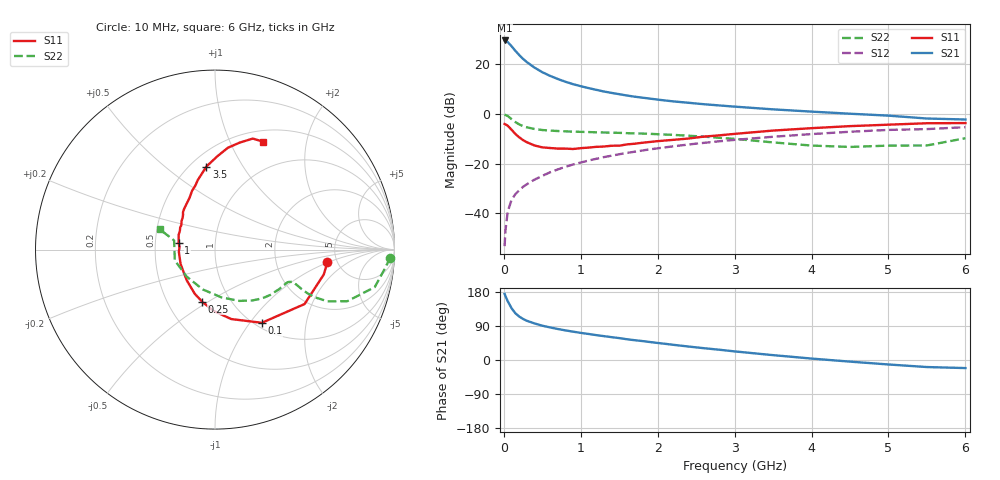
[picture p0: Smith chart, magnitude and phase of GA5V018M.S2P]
! Infineon Technologies  Discrete & RF Semiconductors
! BF775
! Si NPN RF Bipolar Junction Transistor in SOT23
! VCE = 5 V  IC = 18 mA
! Common Emitter S-Parameters:  May  1996
# GHz  S  MA  R  50
!  f  S11  S21  S12  S22
! GHz  MAG  ANG  MAG  ANG  MAG  ANG  MAG  ANG
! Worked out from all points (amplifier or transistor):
!   36 points, 10 MHz to 6 GHz, reference 50 ohm
!   highest |S21| = 29.6 dB at 10 MHz (marker M1)
!   |S21| within 3 dB of that: start of sweep to 118.7 MHz
!   unconditionally stable (mu >= 1): 437.1 MHz to 2.916 GHz
!   at 250 MHz: K = 0.82, MSG = 25.7 dB, |S12| = -29.3 dB
!   at 1.4 GHz: K = 1.10, MAG = 10.7 dB, |S12| = -16.8 dB
!   at 6 GHz: K = 0.93, MSG = 1.5 dB, |S12| = -5.3 dB
!   S11 on the Smith chart (normalised r, x): 10 MHz: 4.16, -0.99; 100 MHz: 1.07, -1.14; 250 MHz: 0.74, -0.47; 1 GHz: 0.66, +0.05; 3.5 GHz: 0.60, +0.71; 6 GHz: 0.63, +1.34
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0.01  0.6304 -6.5  30.22 174.5  0.0022 85.6  0.9769 -2.6
0.02  0.6217 -12.9  29.92 169.3  0.0044 83.9  0.9576 -5.6
0.05  0.5839 -31.3  28.12 155.3  0.0108 77.2  0.9143 -13.2
0.1  0.4841 -57.4  23.17 136.8  0.0188 70.0  0.7915 -21.3
0.15  0.3972 -76.9  18.72 123.3  0.0245 65.6  0.6903 -24.7
0.2  0.3408 -91.6  15.39 114.7  0.0293 65.2  0.6193 -25.5
0.25  0.2986 -103.9  12.88 108.3  0.0344 66.0  0.5713 -25.3
0.3  0.2708 -114.6  11.06 103.4  0.0388 67.2  0.5401 -24.8
0.4  0.2328 -132.4  8.572 96.4  0.0481 68.3  0.5003 -23.5
0.5  0.2138 -146.1  6.946 90.5  0.0571 69.4  0.477 -22.8
0.6  0.2075 -157.5  5.872 86.0  0.0672 69.5  0.4648 -22.8
0.7  0.2019 -167.4  5.082 81.9  0.0768 69.9  0.4558 -23.2
0.8  0.2018 -176.8  4.468 78.2  0.0867 69.4  0.4485 -23.7
1  0.2061 169.5  3.631 71.6  0.106 68.6  0.4385 -25.3
1.1  0.2113 163.2  3.33 68.8  0.1159 68.0  0.434 -26.7
1.3  0.2219 151.8  2.841 63.0  0.136 66.5  0.4259 -29.2
1.6  0.2451 139.5  2.36 54.8  0.1652 63.9  0.4128 -33.7
2.2  0.3026 121.1  1.799 40.2  0.2241 58.0  0.3813 -44.7
3.5  0.4653 95.9  1.243 12.8  0.3493 42.6  0.2689 -82.2
4.5  0.5717 82.8  1.016 -4.3  0.4407 29.5  0.218 -136.2
5.5  0.6534 71.2  0.813 -18.6  0.4981 14.5  0.2334 167.4
6  0.6584 65.9  0.777 -21.3  0.5442 10.3  0.3266 159.9
